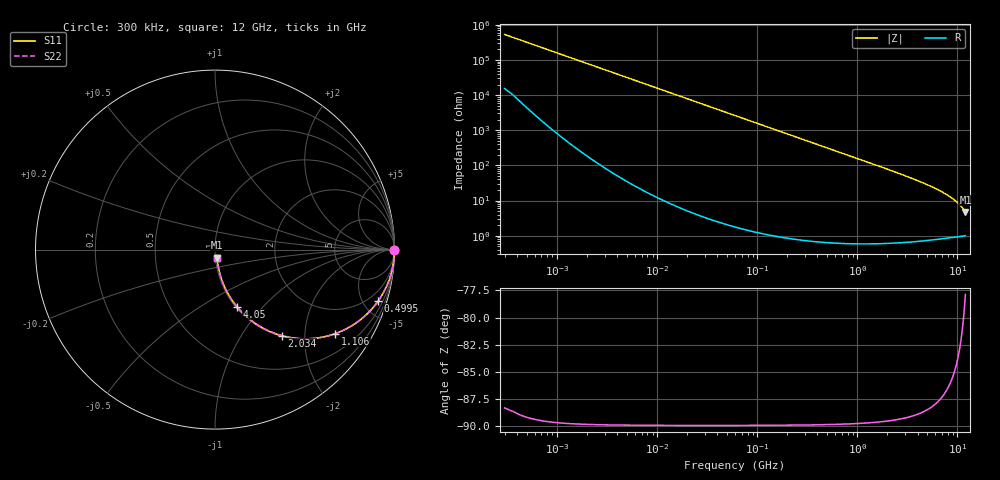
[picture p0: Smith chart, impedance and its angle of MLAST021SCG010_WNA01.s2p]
! MLAST021SCG010_WNA01  S-PARAMETER MODEL  ( General Type )
! Model Generated by TAIYO YUDEN Corporation (http://www.ty-top.com)
! Version 1.0
! TAIYO YUDEN Control No. 220901
! Copyright(c) 2022 TAIYO YUDEN CO.,LTD. All Rights Reserved.
! Product Description (link to TY-COMPAS)
! https://ds.yuden.co.jp/TYCOMPAS/or/detail?pn=MLAST021SCG010BWNA01&u=M
! Products Name : Multilayer Ceramic Capacitors
! Characteristics :
!  Capacitance : 1 pF , Rated Voltage : 25V , TCC : CG / C0G
!  Case Size : 0.25 x 0.125 / 0.0098 x 0.0049 [mm/inch] , Thickness : 0.125 / 0.0049 [mm/inch]
!  (Conditions: Temperature = 25 degC , DC Bias Current/Voltage = 0A / 0V)
! External Node Assignments :
!  1  o---| |---o  2
! GND o---------o GND
! Frequency Range : 0.3MHz  -  12000MHz  [ 401 STEP ]
# MHz S RI R 50
! Freq[MHz].  S11 Real  S11 Imag  S21 Real  S21 Imag  S12 Real  S12 Imag  S22 Real  S22 Imag
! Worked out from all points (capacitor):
!   401 points, 300 kHz to 12 GHz, reference 50 ohm
!   read as one part in series: C = 1 pF near 316.3 kHz
!   lowest |Z| = 4.78 ohm at 12 GHz (marker M1)
!   S11 on the Smith chart (normalised r, x): 300 kHz: open; 499.5 MHz: 1.01, -6.37; 1.106 GHz: 1.01, -2.86; 2.034 GHz: 1.01, -1.54; 4.05 GHz: 1.01, -0.73; 12 GHz: 1.02, -0.09
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0.3  1 -0.000188  5.48e-06 0.000188  5.48e-06 0.000188  1 -0.000188
1.769972  1 -0.00111  4.15e-06 0.00111  4.15e-06 0.00111  1 -0.00111
10.44266  1 -0.00656  4.8e-05 0.00656  4.8e-05 0.00656  1 -0.00656
60  0.9986 -0.0376  0.00144 0.0376  0.00144 0.0376  0.9986 -0.0376
159.8975  0.9899 -0.0995  0.0101 0.0995  0.0101 0.0995  0.9899 -0.0995
244.3004  0.9768 -0.1499  0.0232 0.1499  0.0232 0.1499  0.9768 -0.1499
353.9943  0.9525 -0.2119  0.0475 0.2119  0.0475 0.2119  0.9525 -0.2119
499.5319  0.9097 -0.2857  0.0903 0.2857  0.0903 0.2857  0.9097 -0.2857
743.2595  0.8195 -0.3832  0.1805 0.3832  0.1805 0.3832  0.8195 -0.3832
1105.905  0.6713 -0.4677  0.3287 0.4677  0.3287 0.4677  0.6713 -0.4677
1519.776  0.5177 -0.4968  0.4823 0.4968  0.4823 0.4968  0.5177 -0.4968
2033.931  0.3719 -0.4794  0.6281 0.4794  0.6281 0.4794  0.3719 -0.4794
2088.533  0.3593 -0.4758  0.6407 0.4758  0.6407 0.4758  0.3593 -0.4758
2947.191  0.2151 -0.4047  0.7849 0.4047  0.7849 0.4047  0.2151 -0.4047
4050.141  0.1216 -0.3175  0.8784 0.3175  0.8784 0.3175  0.1216 -0.3175
5868.704  0.0564 -0.2146  0.9436 0.2146  0.9436 0.2146  0.0564 -0.2146
7854.144  0.0289 -0.141  0.9711 0.141  0.9711 0.141  0.0289 -0.141
8732.115  0.0226 -0.116  0.9774 0.116  0.9774 0.116  0.0226 -0.116
9708.23  0.0177 -0.0919  0.9823 0.0919  0.9823 0.0919  0.0177 -0.0919
10511.28  0.015 -0.0743  0.985 0.0743  0.985 0.0743  0.015 -0.0743
11380.75  0.013 -0.057  0.987 0.057  0.987 0.057  0.013 -0.057
12000  0.012 -0.0457  0.988 0.0457  0.988 0.0457  0.012 -0.0457
